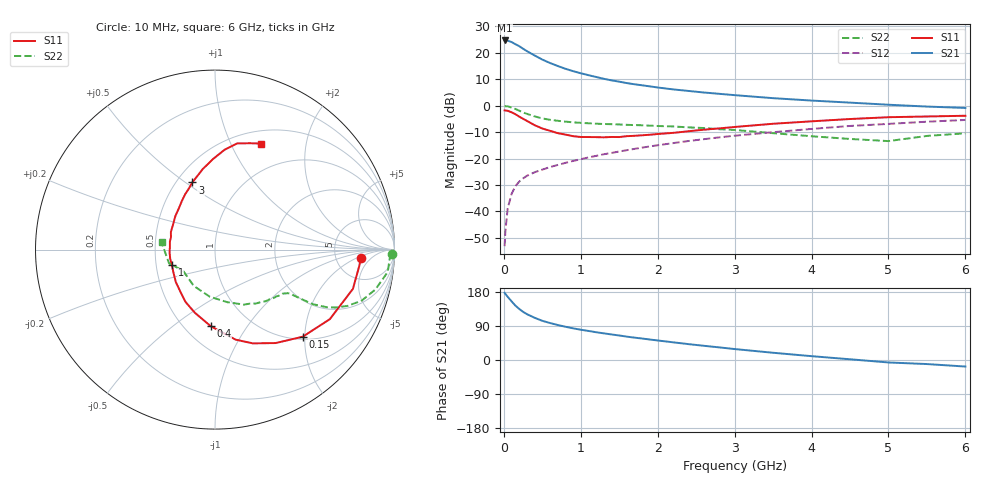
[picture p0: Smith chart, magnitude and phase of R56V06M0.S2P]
! SIEMENS Small Signal Semiconductors
! BFR183
! Si NPN RF Bipolar Junction Transistor in SOT23
! VCE = 6 V  IC = 6 mA
! Common Emitter S-Parameters:  May  1996
# GHz  S  MA  R  50
!  f  S11  S21  S12  S22
! GHz  MAG  ANG  MAG  ANG  MAG  ANG  MAG  ANG
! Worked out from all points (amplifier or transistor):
!   36 points, 10 MHz to 6 GHz, reference 50 ohm
!   highest |S21| = 24.6 dB at 10 MHz (marker M1)
!   |S21| within 3 dB of that: start of sweep to 243.5 MHz
!   unconditionally stable (mu >= 1): 973.5 MHz to 2.634 GHz
!   at 250 MHz: K = 0.46, MSG = 24.5 dB, |S12| = -27.5 dB
!   at 1.4 GHz: K = 1.06, MAG = 12.3 dB, |S12| = -17.9 dB
!   at 6 GHz: K = 0.88, MSG = 2.3 dB, |S12| = -5.4 dB
!   lowest NFmin = 1.20 dB at 450 MHz
!   S11 on the Smith chart (normalised r, x): 10 MHz: 9.10, -2.46; 150 MHz: 1.06, -1.95; 400 MHz: 0.66, -0.69; 1 GHz: 0.61, -0.11; 3 GHz: 0.60, +0.53; 6 GHz: 0.65, +1.31
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0.01  0.8143 -3.2  17.08 177.3  0.0022 94.6  0.9874 -1.4
0.02  0.8091 -6.4  16.82 174.4  0.0042 92.0  0.9747 -2.9
0.05  0.799 -15.9  16.87 166.8  0.0114 80.4  0.9704 -7.4
0.1  0.748 -31.2  15.96 154.9  0.0213 75.1  0.9205 -14.0
0.15  0.6888 -44.8  14.52 143.6  0.03 69.1  0.865 -19.2
0.2  0.6208 -57.0  13.3 134.7  0.0366 64.9  0.8027 -23.0
0.25  0.5635 -68.0  11.92 127.1  0.042 61.6  0.7443 -25.7
0.3  0.5147 -77.1  10.71 121.0  0.0471 60.3  0.6996 -27.3
0.4  0.4273 -93.2  8.89 111.4  0.055 58.3  0.6261 -29.1
0.5  0.3691 -107.8  7.426 103.4  0.0617 58.0  0.573 -29.6
0.6  0.3346 -119.4  6.399 97.6  0.0688 58.2  0.5395 -29.9
0.8  0.2832 -140.5  4.976 87.8  0.0827 58.8  0.4985 -30.3
1  0.2552 -160.0  4.095 79.9  0.0969 60.4  0.4727 -30.9
1.1  0.2548 -168.5  3.768 76.7  0.1049 60.7  0.4638 -31.8
1.3  0.2516 176.7  3.218 70.3  0.1204 60.7  0.4494 -33.2
1.6  0.2648 158.1  2.666 61.6  0.1439 60.0  0.4334 -36.7
2.2  0.3053 131.3  2.028 46.7  0.1955 57.5  0.4037 -45.4
3  0.3947 108.7  1.579 28.9  0.2698 50.8  0.3468 -62.1
3.5  0.4542 98.6  1.384 19.1  0.3146 45.3  0.3013 -76.7
4.5  0.5582 84.6  1.14 1.9  0.4127 33.5  0.2343 -120.3
5.5  0.6235 71.9  0.96 -10.7  0.4966 21.5  0.2674 -163.5
6  0.6436 66.6  0.904 -17.3  0.5358 13.6  0.2998 172.4
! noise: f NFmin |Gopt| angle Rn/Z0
0.45  1.2  0.21  41  0.24
0.9  1.25  0.24  101  0.21
1.8  2  0.32  175  0.14
